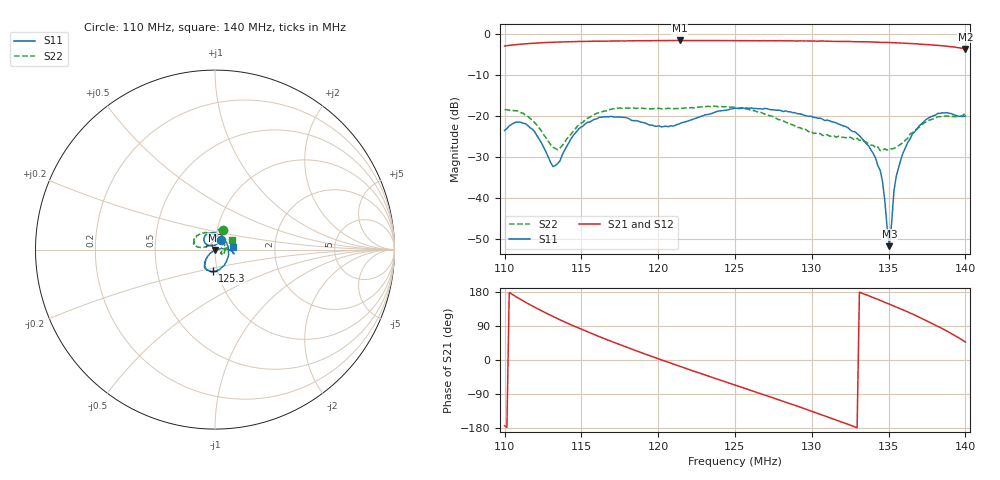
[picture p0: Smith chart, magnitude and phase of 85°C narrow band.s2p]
!Agilent Technologies,E8362C,SG49020144,A.09.33.09
!Agilent E8362C: A.09.33.09
!Date: Friday, October 10, 2025 09:07:54
!Correction: S11(Full 2 Port(1,2))
!S21(Full 2 Port(1,2))
!S12(Full 2 Port(1,2))
!S22(Full 2 Port(1,2))
!S2P File: Measurements: S11, S21, S12, S22:
# Hz S  dB  R 50
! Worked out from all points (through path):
!   201 points, 110 MHz to 140 MHz, reference 50 ohm
!   highest |S21| = -1.66 dB at 121.4 MHz (marker M1); lowest = -3.7 dB at 140 MHz (marker M2)
!   lowest |S11| = -51.8 dB at 135.1 MHz (marker M3), VSWR 1.01, Z = 50.2 - j0.173 ohm
!   |S11| at or under -10 dB: start of sweep to end of sweep
!   |S22| runs from -28.5 to -17.7 dB; largest |S21 - S12| = 0.0067
!   S11 on the Smith chart (normalised r, x): 110 MHz: 1.07, +0.12; 125.3 MHz: 0.95, -0.23; 140 MHz: 1.22, +0.04
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1.1e8  -23.63 57.3  -3.01 -173.6  -3.02 -173.8  -18.54 68.6
1.1135e8  -21.94 62.2  -2.49 152.6  -2.47 152.5  -19.86 80.3
1.1195e8  -23.89 59.5  -2.32 139.3  -2.33 139.3  -21.67 81.2
1.1315e8  -32.42 97.9  -2.09 114.8  -2.11 114.8  -27.68 112.8
1.136e8  -31.05 128.5  -2.03 106.1  -2.04 106.1  -27.90 137.6
1.151e8  -22.57 141.6  -1.88 79.3  -1.88 79.2  -21.61 171.1
1.1765e8  -20.39 98.5  -1.77 38.3  -1.79 38.4  -18.23 164.3
1.2005e8  -22.47 28.9  -1.70 2.7  -1.68 2.8  -18.21 161.5
1.214e8  -21.96 -18.2  -1.66 -16.5  -1.69 -16.6  -18.21 161.5
1.25e8  -18.15 -92.2  -1.69 -66.1  -1.70 -66.2  -17.94 141.7
1.253e8  -18.28 -95.7  -1.70 -70.2  -1.69 -70.2  -18.11 137.7
1.2785e8  -18.66 -117.6  -1.71 -105.1  -1.75 -105.1  -20.98 99.1
1.301e8  -20.41 -125.9  -1.79 -136.7  -1.82 -136.5  -24.32 41.8
1.328e8  -23.89 -134.6  -1.97 -176.5  -1.97 -176.5  -25.94 -24.9
1.34e8  -29.23 -141.7  -2.03 164.7  -2.06 164.8  -27.25 -34.6
1.346e8  -35.97 -139.3  -2.12 155.2  -2.16 155.1  -28.47 -27.0
1.3505e8  -51.83 -42.3  -2.17 147.7  -2.18 147.4  -28.12 -17.6
1.3535e8  -38.28 1.5  -2.20 142.3  -2.22 142.4  -27.98 -9.6
1.355e8  -34.73 6.1  -2.23 139.9  -2.24 140.0  -27.66 -7.0
1.3655e8  -24.41 3.5  -2.42 121.4  -2.41 121.3  -24.16 7.6
1.3835e8  -19.46 -11.4  -2.90 86.0  -2.91 85.8  -20.24 5.7
1.4e8  -20.08 9.3  -3.70 47.5  -3.70 47.4  -19.35 30.6
